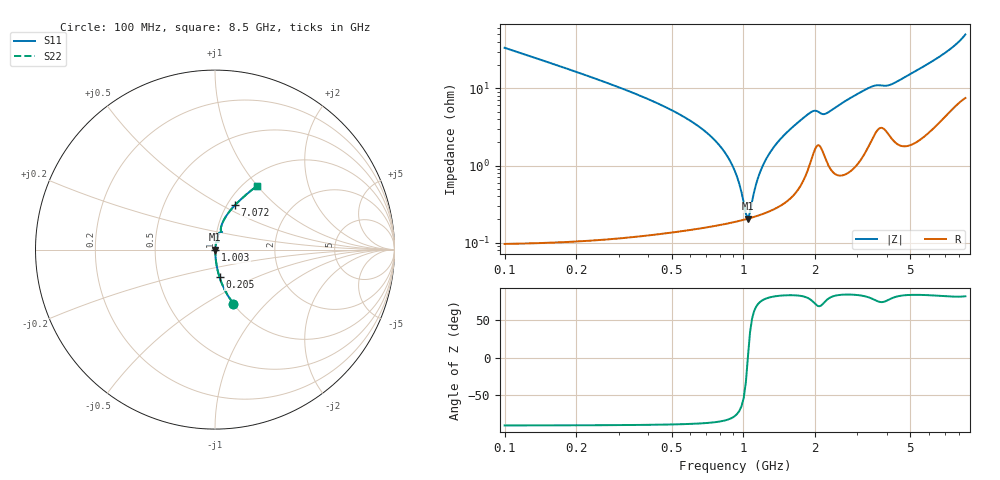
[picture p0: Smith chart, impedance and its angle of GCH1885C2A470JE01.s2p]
!Murata Part Number: GCH1885C2A470JE01
!These Parameters are Measured in Series Mode Connection
!Data Generated on Jun 19, 2026
!  o--ll--o
!Port1  Port2
!  o------o
!Operation Temp=25[degC], DC Bias Voltage=0[V]
!Freq. Start=100[MHz] Stop=9[GHz] 401[Steps]
# Hz S RI R 50
!Freq.(Hz) S11(Real) S11(Imag) S21(Real) S21(Imag) S12(Real) S12(Imag) S22(Real) S22(Imag)
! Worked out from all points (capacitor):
!   401 points, 100 MHz to 8.5 GHz, reference 50 ohm
!   read as one part in series: C = 47 pF near 142 MHz
!   lowest |Z| = 205 mohm at 1.045 GHz (marker M1)
!   series resonance near 1.044 GHz, so ESL is about 490 pH
!   S11 on the Smith chart (normalised r, x): 100 MHz: 1.00, -0.67; 205 MHz: 1.00, -0.32; 1.003 GHz: 1.00, -0.01; 7.072 GHz: 1.09, +0.59; 8.5 GHz: 1.15, +0.99
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1e8  0.1019 -0.301  0.8981 0.301  0.8981 0.301  0.1019 -0.301
2.05e8  0.0256 -0.1546  0.9744 0.1546  0.9744 0.1546  0.0256 -0.1546
3.94e8  0.00662 -0.0732  0.9934 0.0732  0.9934 0.0732  0.00662 -0.0732
6.67e8  0.00244 -0.0301  0.9976 0.0301  0.9976 0.0301  0.00244 -0.0301
7.93e8  0.00202 -0.0182  0.998 0.0182  0.998 0.0182  0.00202 -0.0182
9.19e8  0.00192 -0.00837  0.9981 0.00837  0.9981 0.00837  0.00192 -0.00837
1.003e9  0.00198 -0.00262  0.998 0.00262  0.998 0.00262  0.00198 -0.00262
1.045e9  0.00204 7.72e-05  0.998 -7.72e-05  0.998 -7.72e-05  0.00204 7.72e-05
1.087e9  0.00212 0.00268  0.9979 -0.00268  0.9979 -0.00268  0.00212 0.00268
1.171e9  0.00233 0.00766  0.9977 -0.00766  0.9977 -0.00766  0.00233 0.00766
1.234e9  0.00254 0.0112  0.9975 -0.0112  0.9975 -0.0112  0.00254 0.0112
1.36e9  0.00308 0.0181  0.9969 -0.0181  0.9969 -0.0181  0.00308 0.0181
1.507e9  0.00401 0.0258  0.996 -0.0258  0.996 -0.0258  0.00401 0.0258
1.927e9  0.0141 0.0468  0.9859 -0.0468  0.9859 -0.0468  0.0141 0.0468
2.2e9  0.0143 0.0438  0.9857 -0.0438  0.9857 -0.0438  0.0143 0.0438
2.914e9  0.0154 0.0778  0.9846 -0.0778  0.9846 -0.0778  0.0154 0.0778
3.481e9  0.0323 0.0986  0.9677 -0.0986  0.9677 -0.0986  0.0323 0.0986
4.3e9  0.0324 0.1104  0.9676 -0.1104  0.9676 -0.1104  0.0324 0.1104
5.707e9  0.0564 0.1774  0.9436 -0.1774  0.9436 -0.1774  0.0564 0.1774
7.072e9  0.1124 0.2488  0.8876 -0.2488  0.8876 -0.2488  0.1124 0.2488
7.114e9  0.1147 0.2512  0.8853 -0.2512  0.8853 -0.2512  0.1147 0.2512
8.5e9  0.2318 0.3527  0.7682 -0.3527  0.7682 -0.3527  0.2318 0.3527
